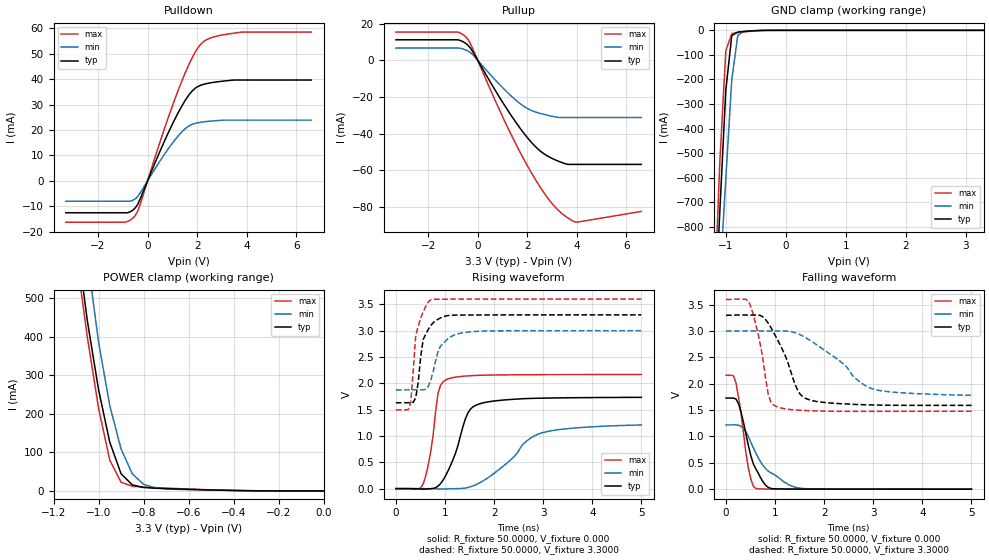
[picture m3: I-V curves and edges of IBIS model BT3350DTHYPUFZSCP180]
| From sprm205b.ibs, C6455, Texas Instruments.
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|   Model BT3350DTHYPUFZSCP180
[Model]   BT3350DTHYPUFZSCP180
Model_type   I/O
Polarity   Non-Inverting
Enable   Active-Low
Vinl =   0.8000V
Vinh =   2.0000V
Vmeas =   1.5000V
Cref =  10.0000pF
Rref =  50.0000
Vref =   1.5000V
C_comp   1.3654pF   1.3131pF   1.4367pF
[Temperature Range]   25.0000   0.1250k   -40.0000
[Pullup Reference]   3.3000V   3.0000V   3.6000V
[Pulldown Reference]   0.000V   0.000V   0.000V
[POWER Clamp Reference]   3.3000V   3.0000V   3.6000V
[GND Clamp Reference]   0.000V   0.000V   0.000V
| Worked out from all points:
|   slope of the pulldown table from 0 to 0.495 V, typ, clamps not added: 42.9 ohm
|   slope of the pullup table from 0 to 0.495 V, typ, clamps not added: 42.8 ohm
|   GND clamp passes 1 mA (typ) near -0.47 V on its own axis
|   POWER clamp passes 1 mA (typ) near -0.38 V on its own axis
|   rising waveform, R_fixture 50.0000, V_fixture 0.000: 20-80 % time 377ps typ, 827ps min, 193ps max; typ from 0 V to 1.73 V
|   rising waveform, R_fixture 50.0000, V_fixture 3.3000: 20-80 % time 182ps typ, 259ps min, 160ps max; typ from 1.63 V to 3.3 V
|   falling waveform, R_fixture 50.0000, V_fixture 0.000: 20-80 % time 305ps typ, 569ps min, 193ps max; typ from 1.73 V to 0 V
|   falling waveform, R_fixture 50.0000, V_fixture 3.3000: 20-80 % time 454ps typ, 923ps min, 247ps max; typ from 3.3 V to 1.59 V
[Pulldown]
| voltage   I(typ)   I(min)   I(max)
-3.3V     -12.59mA   -8.027mA   -16.31mA
-800mV    -12.59mA   NA         -16.01mA
-500mV    -10.71mA   -7.129mA   -13.69mA
-300mV    -7.174mA   -4.816mA   -9.34mA
600mV     13.87mA    9.263mA    18.23mA
1.3V      28.03mA    18.4mA     37.29mA
1.6V      32.9mA     21.17mA    44.34mA
1.9V      36.3mA     22.58mA    50.31mA
2.3V      38.1mA     23.27mA    55.11mA
2.7V      38.83mA    23.63mA    56.76mA
3.5V      39.68mA    NA         58.17mA
6.6V      39.68mA    23.89mA    58.57mA
[Pullup]
| voltage   I(typ)   I(min)   I(max)
-3.3V     11.22mA    6.705mA    15.43mA
-800mV    11.22mA    6.705mA    15.43mA
-500mV    9.448mA    5.765mA    13.06mA
-300mV    6.8mA      4.288mA    9.245mA
1V        -22.82mA   -14.89mA   -30.69mA
2V        -42.2mA    -26.3mA    -57.53mA
2.4V      -48.09mA   -28.53mA   -66.74mA
2.8V      -52.15mA   -29.97mA   -74.81mA
3.2V      -54.81mA   -31.07mA   -81.26mA
3.5V      -56.34mA   NA         -84.78mA
3.7V      -56.87mA   NA         -86.64mA
6.6V      -56.87mA   -31.26mA   -82.55mA
[GND_clamp]
| voltage   I(typ)   I(min)   I(max)
-3.3V     -15.87A    -14.34A    -17.08A
-1.2V     -1.264A    -1.455A    -1.162A
-1.1V     -739.6mA   -1.022A    -540mA
-1V       -245.3mA   -606.1mA   -83.52mA
-900mV    -21.48mA   -201.1mA   -13.14mA
-800mV    -7.057mA   -20.67mA   -8.938mA
-700mV    -4.675mA   -4.511mA   -6.36mA
-300mV    -39.14uA   -55.37uA   -60.92uA
3.3V      64.48uA    87.36uA    296.3nA
[POWER_clamp]
| voltage   I(typ)   I(min)   I(max)
-3.3V     13.83A     12.48A     14.95A
-1.1V     665.8mA    853.9mA    613.9mA
-1.05V    441.8mA    607.3mA    399.6mA
-1V       262.7mA    385.8mA    214.7mA
-950mV    126.2mA    221.3mA    79.62mA
-900mV    44.66mA    108.9mA    22.72mA
-850mV    15.65mA    44.49mA    12.15mA
-800mV    8.944mA    17.22mA    9.922mA
-750mV    7.042mA    8.262mA    8.555mA
-650mV    5.002mA    4.149mA    6.078mA
-350mV    702.5uA    800.3uA    625.3uA
0V        337.7nA    1.605uA    434nA
[Ramp]
| variable   typ   min   max
dV/dt_r   1.0401/0.3729n   0.7249/0.8689n   1.3004/0.1915n
dV/dt_f   1.0262/0.4494n   0.7316/0.9643n   1.2725/0.2450n
R_load = 50.0000
[Rising Waveform]
R_fixture = 50.0000
V_fixture = 0.000
V_fixture_min = 0.000
V_fixture_max = 0.000
| time   V(typ)   V(min)   V(max)
0s        36.67uV    32.36uV    66.72uV
555.6ps   -9.559mV   -328.2uV   90.02mV
707.1ps   -1.584mV   -1.502mV   690.4mV
858.6ps   47.17mV    -5.633mV   1.81V
909.1ps   95.16mV    -6.538mV   1.964V
1.061ns   334mV      -4.009mV   2.084V
1.465ns   1.434V     20.39mV    2.141V
1.667ns   1.598V     91.03mV    2.151V
2.929ns   1.717V     1.046V     2.164V
5ns       1.734V     1.208V     2.167V
[Rising Waveform]
R_fixture = 50.0000
V_fixture = 3.3000
V_fixture_min = 3.0000
V_fixture_max = 3.6000
| time   V(typ)   V(min)   V(max)
0s        1.631V     1.874V     1.496V
252.5ps   1.632V     1.875V     1.503V
303ps     1.631V     1.876V     1.642V
404ps     1.729V     1.875V     2.911V
454.5ps   2.021V     1.875V     3.083V
555.6ps   2.834V     1.876V     3.358V
707.1ps   3.096V     2.047V     3.584V
909.1ps   3.242V     2.708V     3.597V
1.263ns   3.296V     2.94V      3.599V
5ns       3.3V       2.999V     3.6V
[Falling Waveform]
R_fixture = 50.0000
V_fixture = 0.000
V_fixture_min = 0.000
V_fixture_max = 0.000
| time   V(typ)   V(min)   V(max)
0s        1.728V     1.22V      2.16V
151.5ps   1.729V     1.22V      2.151V
202ps     1.709V     1.22V      2.019V
303ps     1.467V     1.194V     1.456V
454.5ps   829.6mV    997.6mV    401.4mV
555.6ps   480.3mV    783.8mV    54.56mV
606.1ps   386.1mV    686mV      13.16mV
858.6ps   33.93mV    343.1mV    2.622mV
1.465ns   2.214mV    25.14mV    594uV
5ns       128.7uV    684.5uV    13.34uV
[Falling Waveform]
R_fixture = 50.0000
V_fixture = 3.3000
V_fixture_min = 3.0000
V_fixture_max = 3.6000
| time   V(typ)   V(min)   V(max)
0s        3.3V       3V         3.6V
454.5ps   3.303V     3.003V     3.569V
656.6ps   3.303V     3.003V     2.928V
858.6ps   3.151V     3.002V     1.803V
1.01ns    2.903V     3.002V     1.575V
1.212ns   2.519V     3.001V     1.522V
1.465ns   1.867V     2.949V     1.499V
1.667ns   1.706V     2.849V     1.49V
2.98ns    1.598V     1.904V     1.476V
5ns       1.59V      1.781V     1.479V
